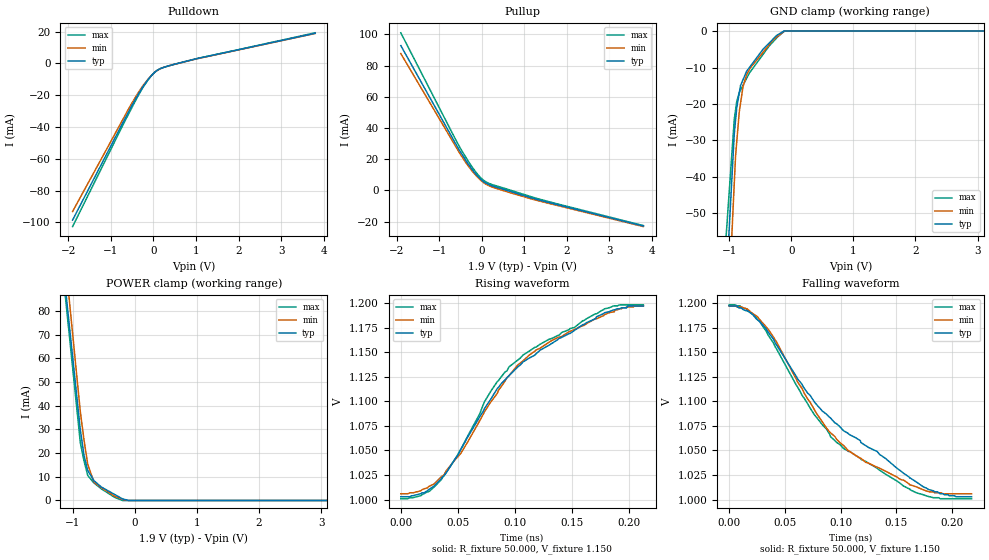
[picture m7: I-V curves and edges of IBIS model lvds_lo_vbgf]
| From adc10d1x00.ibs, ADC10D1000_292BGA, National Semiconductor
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[Model]   lvds_lo_vbgf
Model_type Output
Vref=1.150E+00
Rref=5.000E+01
Cref=0.000E+00
Vmeas=1.150E+00
C_comp   4.84E-13   4.84E-13   4.84E-13
[Voltage Range]   1.900E+00   1.800E+00   2.000E+00
[POWER Clamp Reference]   1.900E+00   1.800E+00   2.000E+00
[GND Clamp Reference]   0.000E+00   0.000E+00   0.000E+00
[Pullup Reference]   1.900E+00   1.800E+00   2.000E+00
[Pulldown Reference]   0.000E+00   0.000E+00   0.000E+00
[Temperature Range]   25   85   -40
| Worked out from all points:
|   slope of the pulldown table from 0 to 0.285 V, typ, clamps not added: 66.9 ohm
|   slope of the pullup table from 0 to 0.285 V, typ, clamps not added: 70.8 ohm
|   GND clamp passes 1 mA (typ) near -0.22 V on its own axis
|   POWER clamp passes 1 mA (typ) near -0.22 V on its own axis
|   rising waveform, R_fixture 50.000, V_fixture 1.150: 20-80 % time 83.6ps typ, 77.8ps min, 75.9ps max; typ from 1 V to 1.2 V
|   falling waveform, R_fixture 50.000, V_fixture 1.150: 20-80 % time 98.4ps typ, 71.4ps min, 79.4ps max; typ from 1.2 V to 1 V
[GND Clamp]
-2V       -371.3mA   -433.9mA   -287.7mA
-1.8V     -307.7mA   -361.3mA   -238.9mA
-920mV    -28.13mA   -41.62mA   -24.12mA
-900mV    -24.54mA   -34.36mA   -21.71mA
-880mV    -20.95mA   -30.31mA   -19.3mA
-840mV    -16.96mA   -22.2mA    -16.87mA
-820mV    -14.96mA   -19.9mA    -16.21mA
-780mV    -13.37mA   -15.3mA    -14.89mA
-720mV    -10.98mA   -11.92mA   -12.92mA
-460mV    -5.066mA   -5.895mA   -6.477mA
-120mV    0A         -127.4uA   -143.4uA
4V        0A         0A         0A
[POWER Clamp]
-2.1V     334mA      361.6mA    336.6mA
-1.7V     234.3mA    255.3mA    234.3mA
-980mV    54.74mA    64.08mA    50.07mA
-880mV    29.81mA    37.52mA    24.48mA
-820mV    19.04mA    25.42mA    16.7mA
-760mV    12.67mA    15.24mA    10.56mA
-660mV    8.358mA    7.751mA    7.391mA
-540mV    5.673mA    5.362mA    4.884mA
-320mV    2.445mA    1.745mA    1.257mA
-200mV    684.9uA    507.8uA    0A
-100mV    0A         0A         0A
3.9V      0A         0A         0A
[Pullup]
-1.9V     92.82mA    87.68mA    101mA
-500mV    24.73mA    23.12mA    26.95mA
-220mV    13.23mA    12.23mA    14.78mA
-100mV    9.243mA    8.547mA    10.42mA
60mV      5.314mA    4.666mA    6.188mA
260mV     2.794mA    1.998mA    3.596mA
1.14V     -4.6mA     -5.285mA   -3.869mA
3.8V      -22.85mA   -23.22mA   -22.58mA
[Pulldown]
-1.9V     -98.51mA   -93.11mA   -102.6mA
-700mV    -36.29mA   -34.3mA    -37.8mA
-480mV    -25.22mA   -23.75mA   -26.35mA
-240mV    -14.38mA   -13.75mA   -14.81mA
-40mV     -7.368mA   -7.302mA   -7.39mA
60mV      -4.874mA   -4.928mA   -4.835mA
260mV     -2.27mA    -2.272mA   -2.281mA
1V        2.931mA    2.834mA    2.969mA
3.8V      19mA       18.87mA    19.29mA
[Rising Waveform]
R_fixture = 50.000
V_fixture = 1.150
V_fixture_min = 1.150
V_fixture_max = 1.150
|  time   V(typ)   V(min)   V(max)
0s        1.003V     1.006V     1.001V
17.5ps    1.006V     1.009V     1.004V
35.25ps   1.021V     1.023V     1.02V
52.5ps    1.051V     1.047V     1.051V
79.25ps   1.103V     1.1V       1.111V
94.75ps   1.126V     1.126V     1.135V
107ps     1.14V      1.141V     1.147V
132.5ps   1.159V     1.162V     1.164V
178.3ps   1.19V      1.188V     1.194V
212.5ps   1.197V     1.197V     1.198V
[Falling Waveform]
R_fixture = 50.000
V_fixture = 1.150
V_fixture_min = 1.150
V_fixture_max = 1.150
|  time   V(typ)   V(min)   V(max)
0s        1.197V     1.197V     1.198V
15.75ps   1.192V     1.194V     1.194V
27.5ps    1.181V     1.183V     1.181V
35.25ps   1.17V      1.173V     1.167V
76.75ps   1.099V     1.091V     1.086V
91ps      1.083V     1.068V     1.064V
106.2ps   1.068V     1.05V      1.05V
168ps     1.018V     1.013V     1.007V
189.2ps   1.006V     1.007V     1.001V
217.5ps   1.003V     1.006V     1.001V
[Ramp]
dV/dt_r   1.7618E+00/8.3350E-11   1.7021E+00/7.6620E-11   1.8224E+00/7.5960E-11
dV/dt_f   1.7618E+00/9.8234E-11   1.7021E+00/7.0641E-11   1.8224E+00/7.9406E-11
R_load = 50
